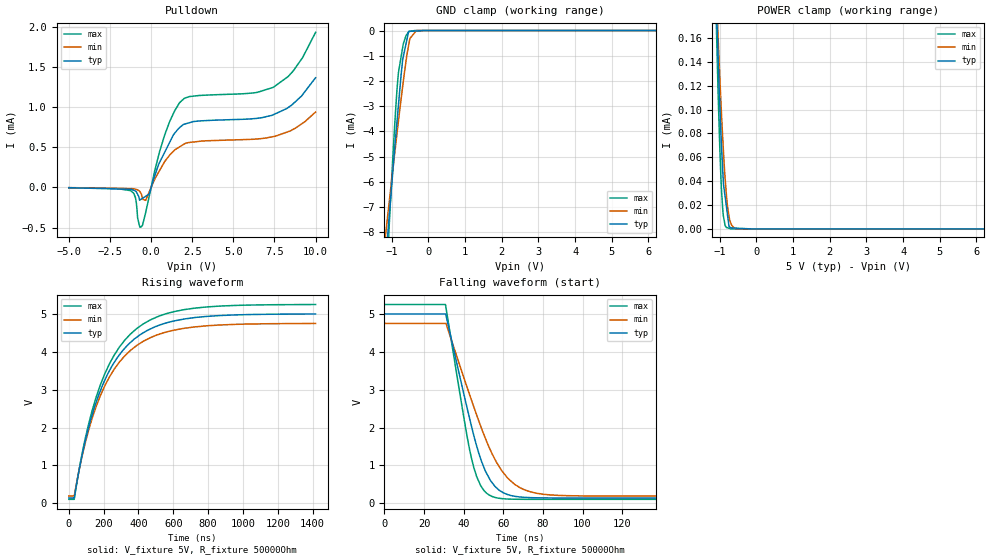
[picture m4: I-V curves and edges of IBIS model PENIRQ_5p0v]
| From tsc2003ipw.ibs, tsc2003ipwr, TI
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[Model]   PENIRQ_5p0v
Model_type   Open_drain
Polarity   Non-Inverting
Enable   Active-High
Vmeas = 2.5
Vref = 2.5
Cref = 1pF
Rref = 50
|   typ   min   max
C_comp   1.404pF   1.208pF   1.903pF
[Voltage Range]   5   4.75   5.25
[Temperature Range]   27   85   -40
[Pullup Reference]   5   4.75   5.25
[Pulldown Reference]   0   0   0
[Power Clamp Reference]   5   4.75   5.25
[GND Clamp Reference]   0   0   0
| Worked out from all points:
|   slope of the pulldown table from 0 to 0.75 V, typ, clamps not added: 1.84 kohm
|   GND clamp passes 1 mA (typ) near -0.68 V on its own axis
|   falling waveform, V_fixture 5V, R_fixture 50000Ohm: 20-80 % time 13.9ns typ, 19.6ns min, 10.2ns max; typ from 5 V to 0.141 V
|   rising waveform, V_fixture 5V, R_fixture 50000Ohm: 20-80 % time 239ns typ, 241ns min, 238ns max; typ from 0.141 V to 5 V
[Pulldown]
|   Voltage   I(typ)   I(min)   I(max)
-5V       -3.261uA   -2.276uA   -5.813uA
-1.234V   -23.27uA   -14.73uA   -40.19uA
-949.3mV  -45.03uA   -22.87uA   -129.7uA
-819.2mV  -85.67uA   -30.95uA   -379.6uA
-613.9mV  -147.4uA   -75.97uA   -492.3uA
-329mV    -110.2uA   -160.7uA   -310uA
-116.9mV  -82.5uA    -57.81uA   -112.6uA
826.6mV   437.4uA    321.1uA    652.9uA
1.727V    742.5uA    503.7uA    1.053mA
7.422V    903.4uA    631.6uA    1.244mA
8.622V    1.038mA    720.2uA    1.444mA
10V       1.364mA    937.5uA    1.929mA
[GND Clamp]
|   Voltage   I(typ)   I(min)   I(max)
-5V       -83.17mA   -60.25mA   -126.4mA
-1.159V   -9.011mA   -7.973mA   -10.25mA
-1.122V   -8.322mA   -7.483mA   -9.185mA
-1.047V   -6.946mA   -6.504mA   -7.083mA
-916.8mV  -4.606mA   -4.831mA   -3.666mA
-819.2mV  -2.975mA   -3.604mA   -1.679mA
-702.3mV  -1.147mA   -2.203mA   -665.4uA
-613.9mV  -541.1uA   -1.24mA    -207.4uA
-540.1mV  -35.19uA   -584.8uA   -53.45uA
-507.1mV  -32.45uA   -320.9uA   -27.94uA
-329mV    -17.64uA   -2.762uA   -161.3nA
10V       0A         0A         0A
[POWER Clamp]
|   Voltage   I(typ)   I(min)   I(max)
-5V       4.857mA    3.977mA    6.567mA
-1.122V   218uA      222.7uA    209uA
-1.047V   147.9uA    164uA      117.8uA
-998.1mV  104.9uA    127.9uA    68.42uA
-949.3mV  68.32uA    94.98uA    31.74uA
-897.3mV  37.61uA    64.67uA    10.42uA
-862.2mV  29.4uA     46.42uA    4.597uA
-819.2mV  19.34uA    29.34uA    1.285uA
-745.7mV  2.138uA    10.34uA    566.1nA
-723.5mV  1.517uA    6.992uA    350nA
-507.1mV  614.1nA    189.7nA    0A
9.985V    0A         0A         0A
[Ramp]
R_load = 50000
|   typ   min   max
dV/dt_r   2.91389/2.39222e-007   2.73249/2.41482e-007   3.08526/2.37843e-007
dV/dt_f   2.91507/1.38618e-008   2.73369/1.95718e-008   3.08639/1.02152e-008
[Falling Waveform]
V_fixture = 5V
V_fixture_min = 4.75V
V_fixture_max = 5.25V
R_fixture = 50000Ohm
C_fixture = 0F
|   Time   V(typ)   V(min)   V(max)
0s        5V         4.75V      5.25V
30.78ns   5V         4.75V      5.247V
41ns      2.681V     3.176V     1.986V
45.07ns   1.8V       2.554V     953.7mV
48.64ns   1.165V     2.031V     461mV
53.48ns   605.1mV    1.407V     203.2mV
61.56ns   244.1mV    709.6mV    115.3mV
74.12ns   149.8mV    298.1mV    106.3mV
103.6ns   141.5mV    195.5mV    106mV
1.417us   141.5mV    193.7mV    106mV
[Rising Waveform]
V_fixture = 5V
V_fixture_min = 4.75V
V_fixture_max = 5.25V
R_fixture = 50000Ohm
C_fixture = 0F
|   Time   V(typ)   V(min)   V(max)
0s        141.5mV    193.7mV    106mV
30.85ns   142.3mV    195mV      106.3mV
92.76ns   1.618V     1.57V      1.682V
133.1ns   2.323V     2.233V     2.437V
181.3ns   2.977V     2.846V     3.13V
260.6ns   3.719V     3.541V     3.913V
388.3ns   4.379V     4.161V     4.607V
540ns     4.735V     4.496V     4.977V
724.7ns   4.904V     4.657V     5.153V
1.417us   4.998V     4.748V     5.248V
